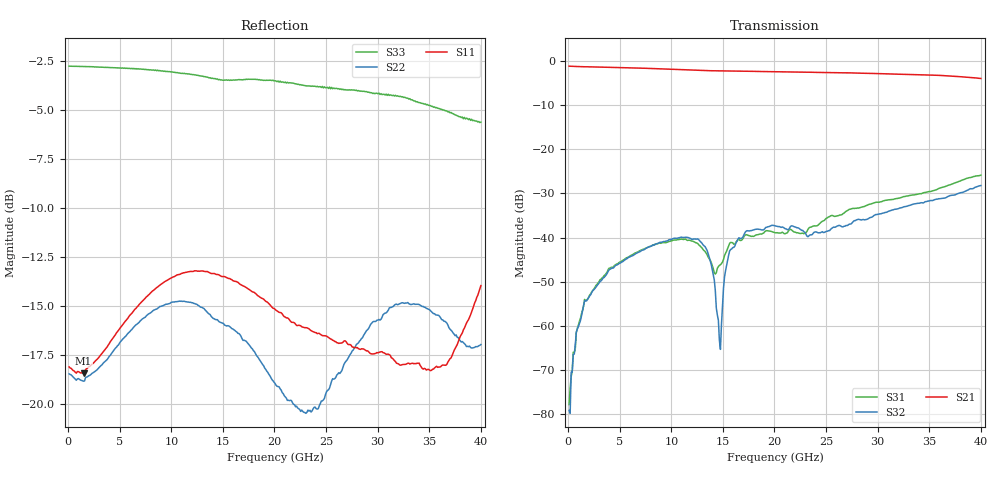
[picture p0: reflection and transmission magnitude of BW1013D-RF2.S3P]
!  3-Port S-parameters saved by WinCal
! VAR MeasName=S-Parameters (CALIBRATED_DATA) read from VNA (N5245A)
! VAR MeasDate=12/26/2016 18:41:52
! VAR NAME=158306_25-RF2
! VAR FILENAME=158306_25-RF2.S3P
! VAR DATE=12/26/2016 18:41:52
! VAR PHYS_PORTS=1,2,3
# Hz S RI R 50
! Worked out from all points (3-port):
!   401 points, 100 MHz to 40 GHz, reference 50 ohm
!   strongest paths, dB at 100 MHz, 10.07 GHz, 20.05 GHz, 30.02 GHz, 40 GHz:
!     S21: -1.2, -1.8, -2.4, -2.8, -3.9
!     S32: -79.2, -40.3, -37.3, -34.7, -28.2
!     S31: -77.8, -40.7, -38.9, -32.0, -25.8
!   lowest |S11| = -18.4 dB at 1.496 GHz (marker M1), VSWR 1.27, Z = 61.4 - j6.91 ohm
!   |S11| at or under -10 dB: start of sweep to end of sweep
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1e8  0.1239 -0.00562  0.8755 -0.0118  0.000123 7.29e-05
     0.8755 -0.0119  0.119 -0.00494  -3.12e-05 3.64e-05
     8.61e-05 9.51e-05  -3.84e-05 0.000103  -0.7277 0.00284
6.985e8  0.1162 -0.0307  0.8661 -0.0737  -0.000206 0.000621
         0.8661 -0.0738  0.1119 -0.0284  -0.00013 0.000639
         -0.000194 0.000517  -0.00016 0.000594  -0.7268 0.0188
1.4965e9  0.1059 -0.0554  0.8494 -0.1461  -0.000111 0.00178
          0.8494 -0.1463  0.1019 -0.0512  -4.6e-05 0.00174
          -0.000169 0.00166  -3.95e-05 0.00169  -0.7252 0.0395
1.157125e10  -0.1247 -0.1774  0.2771 -0.7448  0.00942 0.000396
             0.277 -0.7451  -0.1026 -0.15  0.00995 -0.00296
             0.00926 0.000608  0.00963 -0.0029  -0.6374 0.2781
1.356625e10  -0.1571 -0.1494  0.1274 -0.7681  0.00588 -0.00224
             0.1273 -0.7687  -0.1216 -0.119  0.003 -0.00656
             0.00583 -0.00156  0.00247 -0.00615  -0.604 0.315
1.46635e10  -0.1674 -0.1314  0.0473 -0.7729  0.0041 0.000906
            0.0467 -0.7734  -0.1215 -0.1066  -0.000132 -0.00143
            0.00455 0.00166  -0.000389 -0.000558  -0.586 0.3309
1.576075e10  -0.1734 -0.1145  -0.0349 -0.7712  0.0072 0.00329
             -0.0359 -0.7714  -0.1223 -0.0973  0.00468 0.0044
             0.00801 0.00365  0.00501 0.00537  -0.5753 0.3453
2.005e10  -0.163 -0.0612  -0.3442 -0.6741  0.0113 -0.000731
          -0.3448 -0.6739  -0.0924 -0.0644  0.0118 -0.00533
          0.0113 -0.00122  0.0124 -0.00564  -0.5083 0.4333
3.052375e10  -0.1349 -0.000888  -0.7193 -0.002  0.0163 -0.0206
             -0.7193 -0.00137  -0.0653 -0.1556  0.00736 -0.0171
             0.0162 -0.0203  0.0072 -0.0175  -0.2543 0.5618
4e10  0.1382 0.1448  -0.2843 0.5684  -0.0293 -0.0416
      -0.2833 0.5679  -0.0464 -0.1336  -0.0263 -0.0292
      -0.0293 -0.0417  -0.0263 -0.0287  0.0206 0.5233
